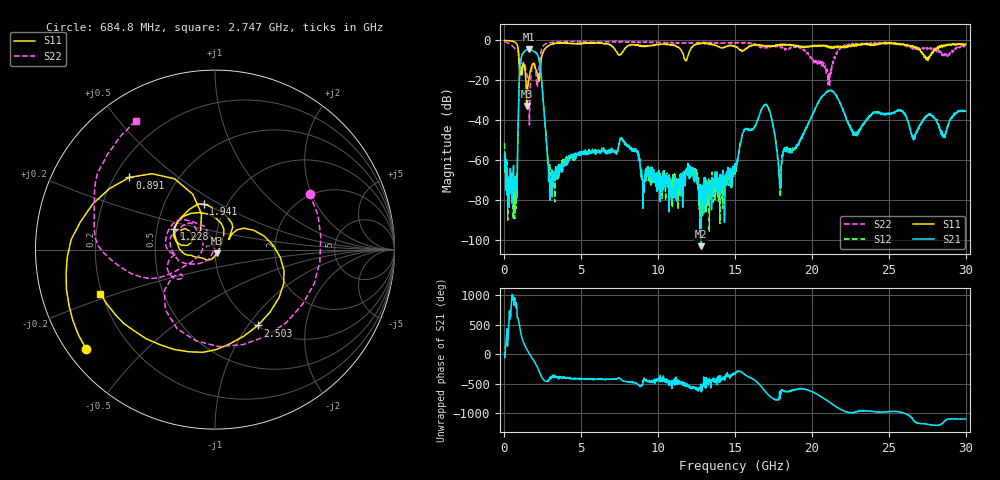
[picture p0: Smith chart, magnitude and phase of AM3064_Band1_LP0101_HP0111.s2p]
# Hz S DB R 50.0
!freq dBS11 angS11 dBS21 angS21 dBS12 angS12 dBS22 angS22
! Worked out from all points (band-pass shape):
!   1600 points, 10 MHz to 29.98 GHz, reference 50 ohm
!   highest |S21| = -4.45 dB at 1.584 GHz (marker M1); lowest = -103.0 dB at 12.79 GHz (marker M2)
!   |S21| within 3 dB of the highest: 1.136 GHz to 2.168 GHz (1.032 GHz wide, 62.4 % of centre)
!   lowest |S11| = -32.8 dB at 1.453 GHz (marker M3), VSWR 1.05, Z = 51 - j2.09 ohm
!   |S11| at or under -10 dB: 949.4 MHz to 2.387 GHz (1.437 GHz wide, 86.2 % of centre); 11.77 GHz to 11.84 GHz (70.83 MHz wide, 0.6 % of centre); 27.52468 GHz to 27.53382 GHz (9.146 MHz wide, 0.0332 % of centre)
!   |S22| runs from -42.3 to -0.3 dB; largest |S21 - S12| = 0.0078
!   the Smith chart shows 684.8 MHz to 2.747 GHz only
!   S11 on the Smith chart (normalised r, x): 684.8 MHz: 0.06, -0.34; 891 MHz: 0.26, +0.34; 1.228 GHz: 0.61, +0.15; 1.941 GHz: 0.78, +0.42; 2.503 GHz: 1.01, -1.12; 2.747 GHz: 0.19, -0.18
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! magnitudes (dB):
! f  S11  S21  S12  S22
! 10 MHz  0.0  -57.0  -51.4  -0.3
! 684.8 MHz  -0.9  -70.2  -68.2  -4.3
! 891 MHz  -4.1  -42.6  -42.5  -6.2
! 1.228 GHz  -11.8  -6.2  -6.2  -11.1
! 1.453 GHz  -32.8  -4.6  -4.6  -16.8
! 1.584 GHz  -19.1  -4.4  -4.5  -27.0
! 1.941 GHz  -11.7  -5.6  -5.5  -12.7
! 2.503 GHz  -6.3  -28.2  -28.1  -3.1
! 2.747 GHz  -3.3  -51.7  -52.3  -1.5
! 3.065 GHz  -1.9  -68.4  -69.0  -1.0
! 5.015 GHz  -1.5  -56.4  -55.6  -0.7
! 7.657 GHz  -6.0  -49.1  -49.2  -0.7
! 10 GHz  -2.1  -69.2  -69.7  -1.0
! 12.79 GHz  -1.5  -103.0  -79.5  -1.1
! 15 GHz  -3.1  -61.7  -64.7  -1.4
! 16.9 GHz  -3.0  -32.4  -32.3  -3.6
! 17.91 GHz  -2.0  -73.4  -67.9  -3.2
! 19.99 GHz  -3.2  -37.8  -37.9  -9.4
! 21.19 GHz  -3.8  -25.0  -24.9  -15.7
! 22.8 GHz  -2.2  -46.5  -47.5  -2.0
! 25 GHz  -1.2  -36.7  -36.6  -1.2
! 29.98 GHz  -1.9  -35.4  -35.3  -2.9
